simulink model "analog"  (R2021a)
settings: Solver=FixedStepDiscrete  StartTime=0.0  StopTime=Inf  RelTol=1e-3  EnableMultiTasking=on
undefined symbols (not defined in the file or in its folder): ADCIN0, ADCIN1, ADCINA0, ADCINB0, bit, ended, input, Single
libraries: c2806xlib x9, c2802xlib x1

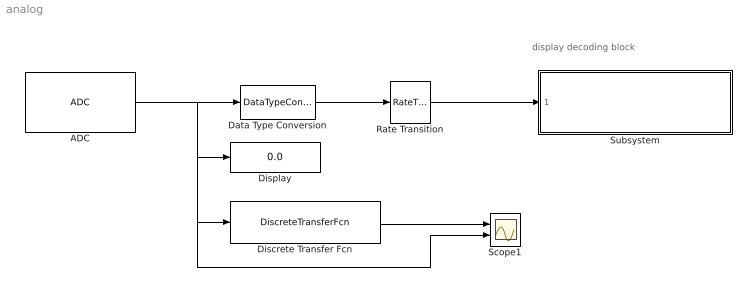
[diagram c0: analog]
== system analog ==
  note: display decoding block
  ADC : c2802xlib/ADC  blkParamProc=C2000  ADCModule=1  samplingMode=Single sample mode  ADCResolution=12-bit (Single-ended input)  useSOC1=SOC0  useSOC2=SOC0_SOC1  SOCAcquisitionWindow=7  SOCTriggerSource=CPU0_TINT0n  SOCInterruptTrigger=No ADCINT  Ts=0.001  dType=single  postInterrupt=off  interruptSel=ADCINT1  ADCINTContinuous=off  endma=off  chdma=1  conv1=ADCINA6  conv2=ADCINA0 and ADCINB0  conv1_Type4=ADCIN0  conv2_Type4=ADCIN0 and ADCIN1
  Data Type Conversion : DataTypeConversion
  Discrete Transfer Fcn : DiscreteTransferFcn  Numerator=[0.003132, 0.003132]  Denominator=[1, -0.9937]
  Display : Display
  Rate Transition : RateTransition
  Scope1 : Scope  NumInputPorts=2
  Subsystem : Subsystem
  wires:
  Data Type Conversion/1 -> Rate Transition/1
  ADC/1 -> Data Type Conversion/1, Discrete Transfer Fcn/1, Scope1/2, Display/1
  Discrete Transfer Fcn/1 -> Scope1/1
  Rate Transition/1 -> Subsystem/1(In1)

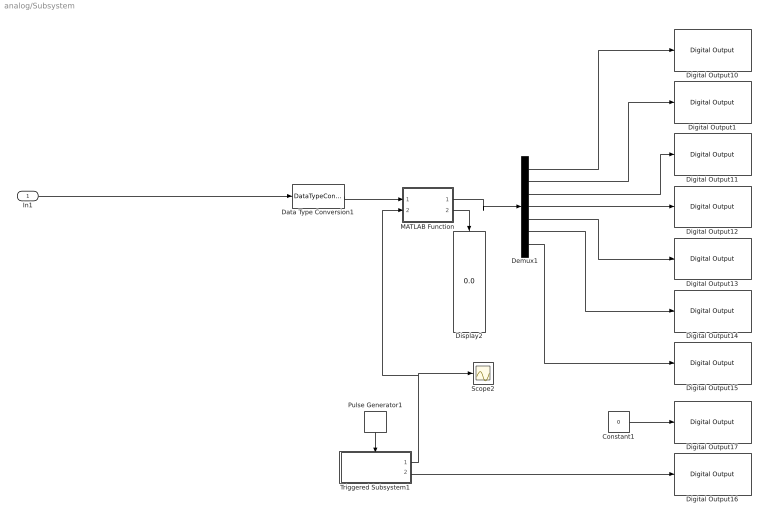
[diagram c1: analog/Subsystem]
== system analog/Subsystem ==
  In1 : Inport
  Constant1 : Constant  Value=0
  Data Type Conversion1 : DataTypeConversion  OutDataTypeStr=uint16
  Demux1 : Demux  Outputs=7
  Digital Output1 : c2806xlib/Digital Output  GPIO_Number=GPIO16~GPIO23  GPIO_Bit0=off  GPIO_BIT0_Toggle=off  GPIO_Bit1=off  GPIO_BIT1_Toggle=off  GPIO_Bit2=off  GPIO_BIT2_Toggle=off  GPIO_Bit3=on  GPIO_BIT3_Toggle=off  GPIO_Bit4=off  GPIO_BIT4_Toggle=off  GPIO_Bit5=off  GPIO_BIT5_Toggle=off  GPIO_Bit6=off  GPIO_BIT6_Toggle=off  GPIO_Bit7=off  GPIO_BIT7_Toggle=off
  Digital Output10 : c2806xlib/Digital Output  GPIO_Number=GPIO50~GPIO55  GPIO_Bit0=off  GPIO_BIT0_Toggle=off  GPIO_Bit1=off  GPIO_BIT1_Toggle=off  GPIO_Bit2=on  GPIO_BIT2_Toggle=off  GPIO_Bit3=off  GPIO_BIT3_Toggle=off  GPIO_Bit4=off  GPIO_BIT4_Toggle=off  GPIO_Bit5=off  GPIO_BIT5_Toggle=off  GPIO_Bit6=off  GPIO_BIT6_Toggle=off  GPIO_Bit7=off  GPIO_BIT7_Toggle=off
  Digital Output11 : c2806xlib/Digital Output  GPIO_Number=GPIO8~GPIO15  GPIO_Bit0=off  GPIO_BIT0_Toggle=off  GPIO_Bit1=off  GPIO_BIT1_Toggle=off  GPIO_Bit2=off  GPIO_BIT2_Toggle=off  GPIO_Bit3=off  GPIO_BIT3_Toggle=off  GPIO_Bit4=off  GPIO_BIT4_Toggle=off  GPIO_Bit5=on  GPIO_BIT5_Toggle=off  GPIO_Bit6=off  GPIO_BIT6_Toggle=off  GPIO_Bit7=off  GPIO_BIT7_Toggle=off
  Digital Output12 : c2806xlib/Digital Output  GPIO_Number=GPIO0~GPIO7  GPIO_Bit0=off  GPIO_BIT0_Toggle=off  GPIO_Bit1=off  GPIO_BIT1_Toggle=off  GPIO_Bit2=off  GPIO_BIT2_Toggle=off  GPIO_Bit3=off  GPIO_BIT3_Toggle=off  GPIO_Bit4=off  GPIO_BIT4_Toggle=off  GPIO_Bit5=on  GPIO_BIT5_Toggle=off  GPIO_Bit6=off  GPIO_BIT6_Toggle=off  GPIO_Bit7=off  GPIO_BIT7_Toggle=off
  Digital Output13 : c2806xlib/Digital Output  GPIO_Number=GPIO16~GPIO23  GPIO_Bit0=off  GPIO_BIT0_Toggle=off  GPIO_Bit1=on  GPIO_BIT1_Toggle=off  GPIO_Bit2=off  GPIO_BIT2_Toggle=off  GPIO_Bit3=off  GPIO_BIT3_Toggle=off  GPIO_Bit4=off  GPIO_BIT4_Toggle=off  GPIO_Bit5=off  GPIO_BIT5_Toggle=off  GPIO_Bit6=off  GPIO_BIT6_Toggle=off  GPIO_Bit7=off  GPIO_BIT7_Toggle=off
  Digital Output14 : c2806xlib/Digital Output  GPIO_Number=GPIO0~GPIO7  GPIO_Bit0=off  GPIO_BIT0_Toggle=off  GPIO_Bit1=off  GPIO_BIT1_Toggle=off  GPIO_Bit2=off  GPIO_BIT2_Toggle=off  GPIO_Bit3=off  GPIO_BIT3_Toggle=off  GPIO_Bit4=on  GPIO_BIT4_Toggle=off  GPIO_Bit5=off  GPIO_BIT5_Toggle=off  GPIO_Bit6=off  GPIO_BIT6_Toggle=off  GPIO_Bit7=off  GPIO_BIT7_Toggle=off
  Digital Output15 : c2806xlib/Digital Output  GPIO_Number=GPIO40~GPIO44  GPIO_Bit0=off  GPIO_BIT0_Toggle=off  GPIO_Bit1=off  GPIO_BIT1_Toggle=off  GPIO_Bit2=off  GPIO_BIT2_Toggle=off  GPIO_Bit3=off  GPIO_BIT3_Toggle=off  GPIO_Bit4=on  GPIO_BIT4_Toggle=off  GPIO_Bit5=off  GPIO_BIT5_Toggle=off  GPIO_Bit6=off  GPIO_BIT6_Toggle=off  GPIO_Bit7=off  GPIO_BIT7_Toggle=off
  Digital Output16 : c2806xlib/Digital Output  GPIO_Number=GPIO0~GPIO7  GPIO_Bit0=on  GPIO_BIT0_Toggle=off  GPIO_Bit1=on  GPIO_BIT1_Toggle=off  GPIO_Bit2=on  GPIO_BIT2_Toggle=off  GPIO_Bit3=on  GPIO_BIT3_Toggle=off  GPIO_Bit4=off  GPIO_BIT4_Toggle=off  GPIO_Bit5=off  GPIO_BIT5_Toggle=off  GPIO_Bit6=off  GPIO_BIT6_Toggle=off  GPIO_Bit7=off  GPIO_BIT7_Toggle=off
  Digital Output17 : c2806xlib/Digital Output  GPIO_Number=GPIO16~GPIO23  GPIO_Bit0=on  GPIO_BIT0_Toggle=off  GPIO_Bit1=off  GPIO_BIT1_Toggle=off  GPIO_Bit2=off  GPIO_BIT2_Toggle=off  GPIO_Bit3=off  GPIO_BIT3_Toggle=off  GPIO_Bit4=off  GPIO_BIT4_Toggle=off  GPIO_Bit5=off  GPIO_BIT5_Toggle=off  GPIO_Bit6=off  GPIO_BIT6_Toggle=off  GPIO_Bit7=off  GPIO_BIT7_Toggle=off
  Display2 : Display
  MATLAB Function : MATLAB Function  TreatAsAtomicUnit=on
  Pulse Generator1 : DiscretePulseGenerator  SampleTime=0.001
  Scope2 : Scope
  Triggered Subsystem1 : Subsystem  TreatAsAtomicUnit=on
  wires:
  Data Type Conversion1/1 -> MATLAB Function/1(num)
  Demux1/2 -> Digital Output1/1
  Triggered Subsystem1/2(digit) -> Digital Output16/1
  Pulse Generator1/1 -> Triggered Subsystem1/Trigger
  MATLAB Function/1(y) -> Demux1/1
  Constant1/1 -> Digital Output17/1
  Triggered Subsystem1/1(n) -> Scope2/1, MATLAB Function/2(digit)
  MATLAB Function/2(w) -> Display2/1
  Demux1/1 -> Digital Output10/1
  Demux1/3 -> Digital Output11/1
  Demux1/5 -> Digital Output13/1
  Demux1/6 -> Digital Output14/1
  Demux1/7 -> Digital Output15/1
  Demux1/4 -> Digital Output12/1
  In1/1 -> Data Type Conversion1/1

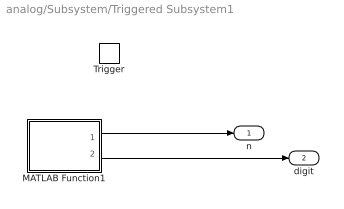
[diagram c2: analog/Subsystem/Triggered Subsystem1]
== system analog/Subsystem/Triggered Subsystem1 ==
  Trigger : TriggerPort  VariantControl=(inherit)
  MATLAB Function1 : MATLAB Function  TreatAsAtomicUnit=on
  n : Outport
  digit : Outport  Port=2
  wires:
  MATLAB Function1/1(nn) -> n/1
  MATLAB Function1/2(digit) -> digit/1

== matlab function analog/Subsystem/Triggered
Subsystem1/MATLAB Function1 ==
function [nn, digit]= fcn


    persistent n

    digit = [1 0 0 0]
        
    if isempty(n)
        n = 0;
    else
        n = n+1;
    end
    
    if n>3
        n=0;
    end
  
    switch n
        case 3
            digit = [0 0 0 1]
        case 2
            digit = [0 0 1 0]
        case 1
            digit = [0 1 0 0]
        case 0
            digit = [1 0 0 0]
    end
    nn=n

y = [nn,digit];

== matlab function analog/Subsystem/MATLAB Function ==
function [y,w]= fcn(num,digit)

  segments = [0 0 0 0 0 0 0]
  x = uint16(0)
  

    
    k   = idivide(num,1000);
    num = num - k*1000;
        
    h  = idivide(num,100);
    num = num - h*100;
        
    da = idivide( num,10 );
    num = num - da*10;
      
    u  = num;
        
        
    switch digit 
        case 0
            % u
            x = u;
        case 1
            % da
            x = da;
        case 2
            % h
            x = h;
        case 3
            % k
            x = k;
            
    end
        
    
switch x
    case 0
        segments = [1 1 1 1 1 1 0]
    case 1
        segments = [0 1 1 0 0 0 0]
    case 2
        segments = [1 1 0 1 1 0 1]
    case 3
        segments = [1 1 1 1 0 0 1]
    case 4
        segments = [0 1 1 0 0 1 1]
    case 5
        segments = [1 0 1 1 0 1 1]
    case 6
        segments = [1 0 1 1 1 1 1]
    case 7
        segments = [1 1 1 0 0 0 0]
    case 8
        segments = [1 1 1 1 1 1 1]
    case 9
        segments = [1 1 1 0 0 1 1]
    otherwise
        segments = [0 0 0 0 0 0 1]

end


y = segments
w = [k h da u];
